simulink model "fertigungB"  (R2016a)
settings: Solver=FixedStepDiscrete  StartTime=0.0  StopTime=25.1  RelTol=1e-3
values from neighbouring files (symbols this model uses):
  dt = block.DialogPrm(4).Data    [sfun_oven.m]
  t0 = block.DialogPrm(5).Data    [sfun_oven.m]
undefined symbols (not defined in the file or in its folder): m0, ndelay
libraries: simulink x1

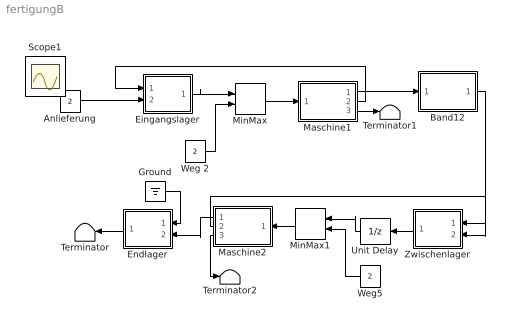
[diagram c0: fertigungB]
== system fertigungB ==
  Anlieferung : Constant  Value=2
  Band12 : Subsystem
  Eingangslager : Subsystem
  Endlager : Subsystem
  Ground : Ground
  Maschine1 : Subsystem
  Maschine2 : Subsystem
  MinMax : MinMax  Inputs=2
  MinMax1 : MinMax  Inputs=2
  Terminator : Terminator
  Terminator1 : Terminator
  Terminator2 : Terminator
  Unit Delay : UnitDelay  SampleTime=-1
  Weg 2 : Constant  Value=2
  Weg5 : Constant  Value=2
  Zwischenlager : Subsystem
  Scope1 : Scope
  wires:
  Anlieferung/1 -> Eingangslager/2(In2)
  MinMax/1 -> Maschine1/1(in)
  Eingangslager/1(Out1) -> MinMax/1
  Weg 2/1 -> MinMax/2
  Maschine1/1(out) -> Band12/1(In)
  MinMax1/1 -> Maschine2/1(in)
  Weg5/1 -> MinMax1/2
  Maschine2/1(out) -> Endlager/2(In2)
  Maschine1/2(increment) -> Eingangslager/1(In1)
  Endlager/1(Out1) -> Terminator/1
  Maschine1/3(load) -> Terminator1/1
  Zwischenlager/1(Out1) -> Unit Delay/1
  Band12/1(Out) -> Zwischenlager/2(In2)
  Maschine2/2(increment) -> Zwischenlager/1(In1)
  Unit Delay/1 -> MinMax1/1
  Maschine2/3(load) -> Terminator2/1
  Ground/1 -> Endlager/1(In1)

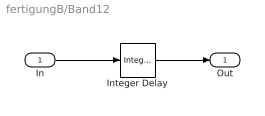
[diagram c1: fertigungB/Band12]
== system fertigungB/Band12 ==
  In : Inport
  Integer Delay : simulink/Discrete/Integer Delay  NumDelays=ndelay  vinit=0.0  samptime=[dt,t0]
  Out : Outport
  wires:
  Integer Delay/1 -> Out/1
  In/1 -> Integer Delay/1

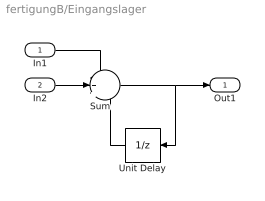
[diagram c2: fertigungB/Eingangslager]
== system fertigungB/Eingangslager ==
  In1 : Inport
  In2 : Inport  Port=2
  Sum : Sum  Inputs=-++
  Unit Delay : UnitDelay  InitialCondition=m0  SampleTime=[dt, t0]
  Out1 : Outport
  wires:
  Unit Delay/1 -> Sum/3
  In2/1 -> Sum/2
  Sum/1 -> Unit Delay/1, Out1/1
  In1/1 -> Sum/1

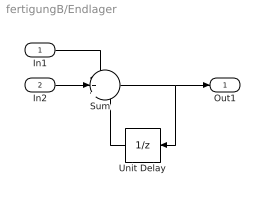
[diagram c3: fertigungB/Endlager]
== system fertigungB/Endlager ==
  In1 : Inport
  In2 : Inport  Port=2
  Sum : Sum  Inputs=-++
  Unit Delay : UnitDelay  InitialCondition=m0  SampleTime=[dt, t0]
  Out1 : Outport
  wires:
  Unit Delay/1 -> Sum/3
  In2/1 -> Sum/2
  Sum/1 -> Unit Delay/1, Out1/1
  In1/1 -> Sum/1

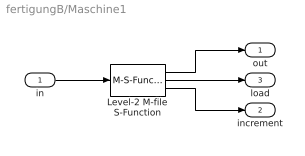
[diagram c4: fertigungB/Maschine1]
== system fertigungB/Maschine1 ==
  in : Inport
  Level-2 M-file S-Function : M-S-Function  FunctionName=sfun_oven  Parameters=capacity, cookingtime, initload, dt, t0
  out : Outport
  increment : Outport  Port=2
  load : Outport  Port=3
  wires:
  Level-2 M-file S-Function/3 -> increment/1
  Level-2 M-file S-Function/2 -> load/1
  Level-2 M-file S-Function/1 -> out/1
  in/1 -> Level-2 M-file S-Function/1

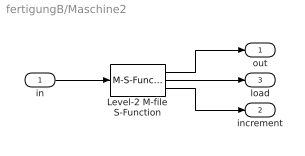
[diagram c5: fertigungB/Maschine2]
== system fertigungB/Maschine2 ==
  in : Inport
  Level-2 M-file S-Function : M-S-Function  FunctionName=sfun_oven  Parameters=capacity, cookingtime, initload, dt, t0
  out : Outport
  increment : Outport  Port=2
  load : Outport  Port=3
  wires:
  Level-2 M-file S-Function/3 -> increment/1
  Level-2 M-file S-Function/2 -> load/1
  Level-2 M-file S-Function/1 -> out/1
  in/1 -> Level-2 M-file S-Function/1

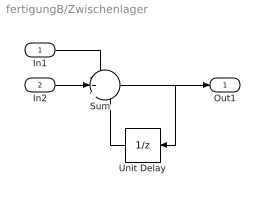
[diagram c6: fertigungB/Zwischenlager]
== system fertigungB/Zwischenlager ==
  In1 : Inport
  In2 : Inport  Port=2
  Sum : Sum  Inputs=-++
  Unit Delay : UnitDelay  InitialCondition=m0  SampleTime=[dt, t0]
  Out1 : Outport
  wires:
  Unit Delay/1 -> Sum/3
  In2/1 -> Sum/2
  Sum/1 -> Unit Delay/1, Out1/1
  In1/1 -> Sum/1
